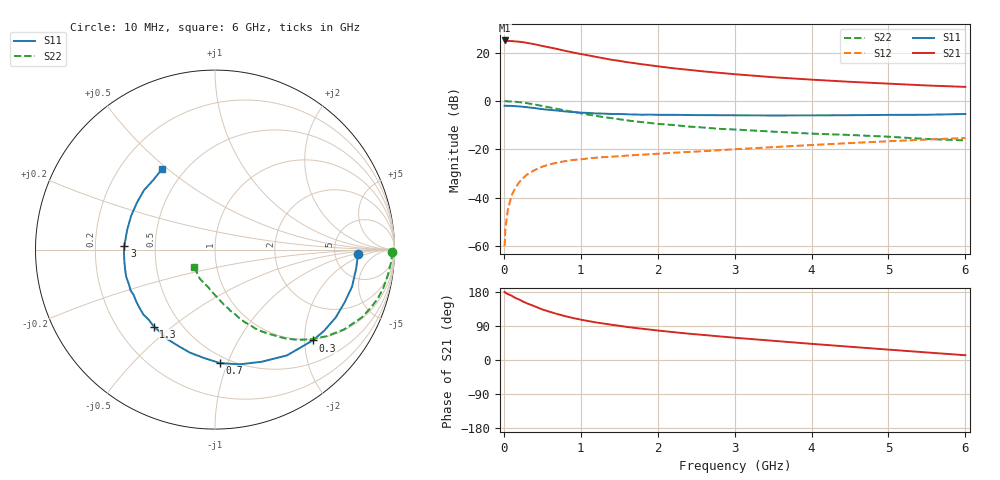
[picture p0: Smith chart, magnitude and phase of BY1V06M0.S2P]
! SIEMENS Small Signal Semiconductors
! BFY420
! Si NPN RF SIEGET Grounded Emitter Transistor in MICRO-X
! VCE = 1 V  IC = 6 mA
! Common Emitter S-Parameters:  October  1996
# GHz  S  MA  R  50
!  f  S11  S21  S12  S22
! GHz  MAG  ANG  MAG  ANG  MAG  ANG  MAG  ANG
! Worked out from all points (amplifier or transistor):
!   36 points, 10 MHz to 6 GHz, reference 50 ohm
!   highest |S21| = 25.0 dB at 10 MHz (marker M1)
!   |S21| within 3 dB of that: start of sweep to 615 MHz
!   unconditionally stable (mu >= 1): 2.869 GHz to end of sweep
!   at 250 MHz: K = 0.12, MSG = 28.1 dB, |S12| = -31.9 dB
!   at 1.4 GHz: K = 0.61, MSG = 20.0 dB, |S12| = -23.0 dB
!   at 6 GHz: K = 1.15, MAG = 8.2 dB, |S12| = -15.3 dB
!   S11 on the Smith chart (normalised r, x): 10 MHz: 8.67, -1.12; 300 MHz: 0.97, -2.18; 700 MHz: 0.45, -0.94; 1.3 GHz: 0.35, -0.43; 3 GHz: 0.33, +0.02; 6 GHz: 0.38, +0.48
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0.01  0.7962 -1.7  17.78 179.8  0.001 81.6  0.9846 -0.8
0.02  0.7958 -3.3  17.75 177.4  0.0022 91.2  0.9876 -1.6
0.05  0.7936 -7.6  17.37 174.2  0.0054 85.3  0.983 -4.3
0.1  0.791 -15.1  17.28 169.8  0.0111 83.3  0.9723 -8.8
0.15  0.7799 -22.1  16.96 163.7  0.0161 77.0  0.9619 -12.9
0.2  0.7715 -29.4  16.75 159.5  0.0209 75.6  0.9465 -17.0
0.25  0.7578 -36.7  16.36 154.2  0.0255 71.5  0.9228 -21.0
0.3  0.7432 -42.9  15.85 149.6  0.03 69.0  0.9012 -24.8
0.4  0.7131 -55.7  14.85 141.7  0.0374 62.7  0.8459 -31.7
0.5  0.677 -67.4  13.69 133.4  0.0439 57.8  0.7884 -37.7
0.6  0.6536 -78.0  12.74 127.0  0.0493 53.7  0.7338 -42.9
0.7  0.6329 -87.5  11.78 121.0  0.0534 50.1  0.6832 -47.4
0.9  0.5909 -103.7  10.02 110.7  0.0605 44.6  0.5922 -54.5
1.1  0.5654 -117.9  8.739 102.7  0.0651 41.5  0.5214 -60.6
1.3  0.5477 -128.5  7.607 96.1  0.0692 39.3  0.4631 -65.0
1.7  0.5252 -146.9  6.033 84.8  0.076 36.8  0.3791 -72.5
2.2  0.5173 -163.2  4.747 73.6  0.085 35.2  0.3187 -79.8
3  0.5057 177.7  3.572 58.8  0.1005 33.2  0.2575 -89.2
3.5  0.5016 166.9  3.095 50.7  0.1113 31.8  0.2322 -95.1
4.5  0.5076 148.9  2.486 35.0  0.1348 26.7  0.1983 -107.4
5.5  0.5188 131.1  2.089 19.9  0.1598 20.0  0.1638 -127.6
6  0.5377 123.2  1.953 12.6  0.1717 16.2  0.1532 -140.8
